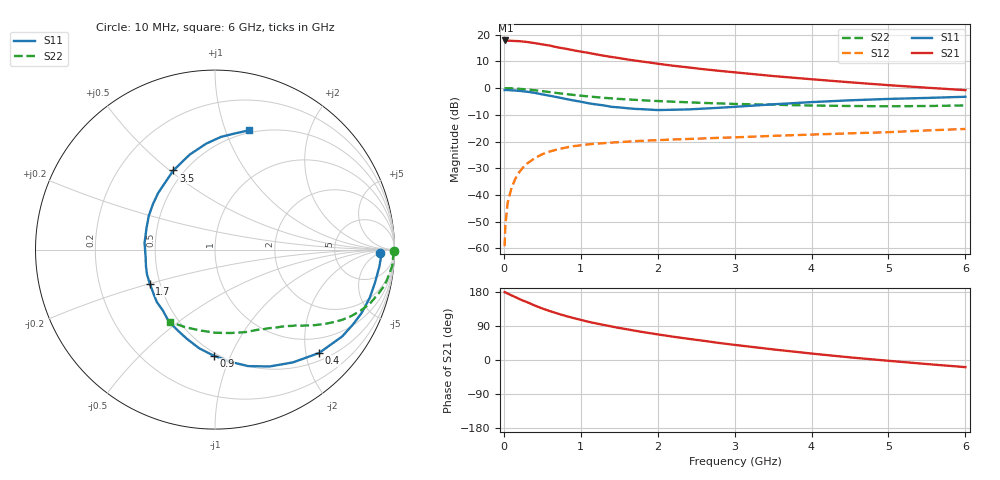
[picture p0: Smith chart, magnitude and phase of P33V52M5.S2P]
! SIEMENS Small Signal Semiconductors
! BFP181
! Si NPN RF Bipolar Junction Transistor in SOT143
! VCE = 3.5 V  IC = 2.5 mA
! Common Emitter S-Parameters:  March  1996
# GHz  S  MA  R  50
!  f  S11  S21  S12  S22
! GHz  MAG  ANG  MAG  ANG  MAG  ANG  MAG  ANG
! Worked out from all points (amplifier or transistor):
!   36 points, 10 MHz to 6 GHz, reference 50 ohm
!   highest |S21| = 17.9 dB at 20 MHz (marker M1)
!   |S21| within 3 dB of that: start of sweep to 782.3 MHz
!   unconditionally stable (mu >= 1): 2.291 GHz to end of sweep
!   at 250 MHz: K = 0.14, MSG = 23.6 dB, |S12| = -29.7 dB
!   at 1.4 GHz: K = 0.71, MSG = 16.0 dB, |S12| = -20.4 dB
!   at 6 GHz: K = 1.11, MAG = 5.2 dB, |S12| = -15.3 dB
!   S11 on the Smith chart (normalised r, x): 10 MHz: 22, -6; 400 MHz: 0.65, -2.27; 900 MHz: 0.48, -0.87; 1.7 GHz: 0.44, -0.20; 3.5 GHz: 0.44, +0.51; 6 GHz: 0.48, +1.21
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0.01  0.9184 -1.3  7.815 179.1  0.0011 83.4  0.9962 -0.5
0.02  0.9256 -2.4  7.818 178.5  0.0027 90.5  0.9952 -1.0
0.05  0.921 -5.8  7.77 175.2  0.0072 87.8  0.9928 -2.7
0.15  0.903 -17.3  7.631 165.9  0.0202 79.0  0.9804 -7.8
0.25  0.8737 -28.8  7.455 156.6  0.0328 73.3  0.9587 -12.8
0.3  0.8582 -34.3  7.325 152.9  0.0385 69.9  0.944 -15.0
0.4  0.8174 -44.8  6.979 143.9  0.0487 64.0  0.9134 -19.3
0.5  0.7641 -55.3  6.596 135.9  0.058 58.8  0.8782 -22.9
0.6  0.7191 -64.9  6.26 128.9  0.0653 54.2  0.8417 -26.3
0.7  0.6754 -74.0  5.802 122.5  0.0715 50.2  0.808 -29.0
0.8  0.6308 -82.3  5.479 116.5  0.0769 46.7  0.7764 -31.3
0.9  0.5909 -90.7  5.145 111.0  0.0819 43.5  0.749 -33.3
1.1  0.5212 -107.5  4.577 100.8  0.0888 38.6  0.7001 -36.9
1.4  0.447 -130.4  3.837 88.5  0.0957 33.3  0.6441 -41.2
1.7  0.4096 -152.5  3.292 77.5  0.1019 30.0  0.6045 -44.7
1.9  0.3957 -166.4  3.012 70.8  0.105 28.0  0.5833 -47.1
2.2  0.3942 174.5  2.632 61.5  0.1094 26.1  0.5579 -50.8
2.8  0.4294 143.4  2.11 44.9  0.1175 23.4  0.5185 -58.9
3.5  0.4983 117.8  1.687 28.0  0.1279 20.5  0.4898 -69.9
4.5  0.5922 94.8  1.287 6.9  0.1426 16.8  0.4635 -89.6
5.5  0.6564 80.3  1.019 -10.7  0.1616 14.0  0.463 -111.0
6  0.6904 74.2  0.918 -18.8  0.1722 11.5  0.4747 -122.0
